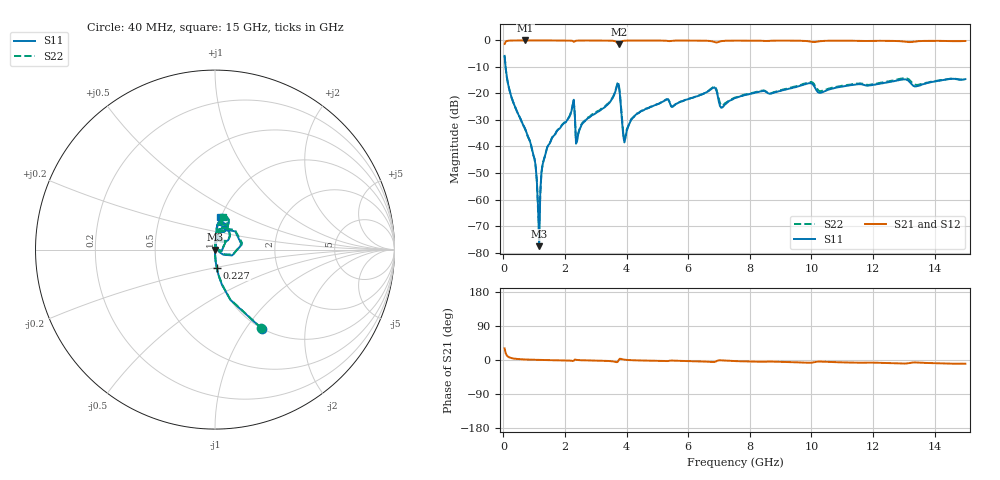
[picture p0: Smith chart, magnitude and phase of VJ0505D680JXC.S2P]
! VJ0505D680JXP
! MLCC placed on 25 mil thick microstrip substrate in series configuraton.
! DATE 06/29/2018  09:34
! CORRECTED  DATA
# GHz  S  MA  R  50.00
!  FREQ  S11M  S11A  S21M  S21A  S12M  S12A  S22M  S22A
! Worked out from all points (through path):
!   401 points, 40 MHz to 15 GHz, reference 50 ohm
!   highest |S21| = -0.02 dB at 713.2 MHz (marker M1); lowest = -1.4 dB at 3.743 GHz (marker M2)
!   group delay of S21, straight-line fit = 2.2 ps
!   lowest |S11| = -77.6 dB at 1.162 GHz (marker M3), VSWR 1.00, Z = 50 + j0.00665 ohm
!   |S11| at or under -10 dB: 72.2 MHz to end of sweep
!   |S22| runs from -69.6 to -5.9 dB; largest |S21 - S12| = 0.0027
!   S11 on the Smith chart (normalised r, x): 40 MHz: 1.00, -1.19; 227 MHz: 1.00, -0.20; 15 GHz: 0.99, +0.38
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0.04  0.511 -59.4  0.859 30.6  0.8602 30.6  0.5068 -59.4
0.227  0.1005 -84.4  0.9934 5.8  0.9939 5.9  0.09943 -84.4
0.7132  0.02104 -89.3  0.9981 1.4  0.9982 1.5  0.02094 -88.3
0.975  0.006868 -92.4  0.998 0.6  0.9982 0.7  0.006764 -91.9
1.0872  0.00218 -91.3  0.9981 0.4  0.9981 0.5  0.002226 -87.7
1.162  0.0001319 149.7  0.9978 0.3  0.9982 0.4  0.0003309 113.5
1.3116  0.005496 90.1  0.9975 0.0  0.9978 0.1  0.005591 90.6
1.536  0.01251 87.6  0.9974 -0.3  0.9974 -0.2  0.01262 87.9
2.2092  0.04654 78.4  0.989 -1.9  0.9888 -1.8  0.04714 79.0
2.4336  0.01745 80.5  0.9942 -0.2  0.9946 -0.1  0.01805 81.1
2.5458  0.02594 86.6  0.9956 -0.7  0.996 -0.6  0.02696 86.3
3.7426  0.1511 10.4  0.8487 -0.7  0.8488 -0.7  0.1552 13.6
3.8922  0.01581 -10.8  0.9811 1.4  0.9809 1.5  0.01806 -6.5
3.967  0.01485 60.7  0.9894 0.5  0.9894 0.6  0.01676 56.1
4.2662  0.03786 86.6  0.9949 -0.8  0.9951 -0.8  0.03795 85.3
5.0516  0.06448 86.6  0.9939 -2.2  0.9941 -2.1  0.06387 86.3
6.8094  0.1279 66.1  0.9516 -5.3  0.9524 -5.3  0.1311 68.3
7.1086  0.05441 66.2  0.974 -1.2  0.9746 -1.1  0.05864 63.9
7.52  0.08205 85.4  0.991 -2.9  0.9916 -2.9  0.08363 84.2
10.0258  0.1521 66.1  0.9398 -6.8  0.9405 -6.8  0.1626 65.7
12.5316  0.1639 80.4  0.9804 -8.2  0.9809 -8.2  0.17 80.6
15  0.1861 81.0  0.9749 -9.9  0.9755 -10.0  0.1877 76.0
